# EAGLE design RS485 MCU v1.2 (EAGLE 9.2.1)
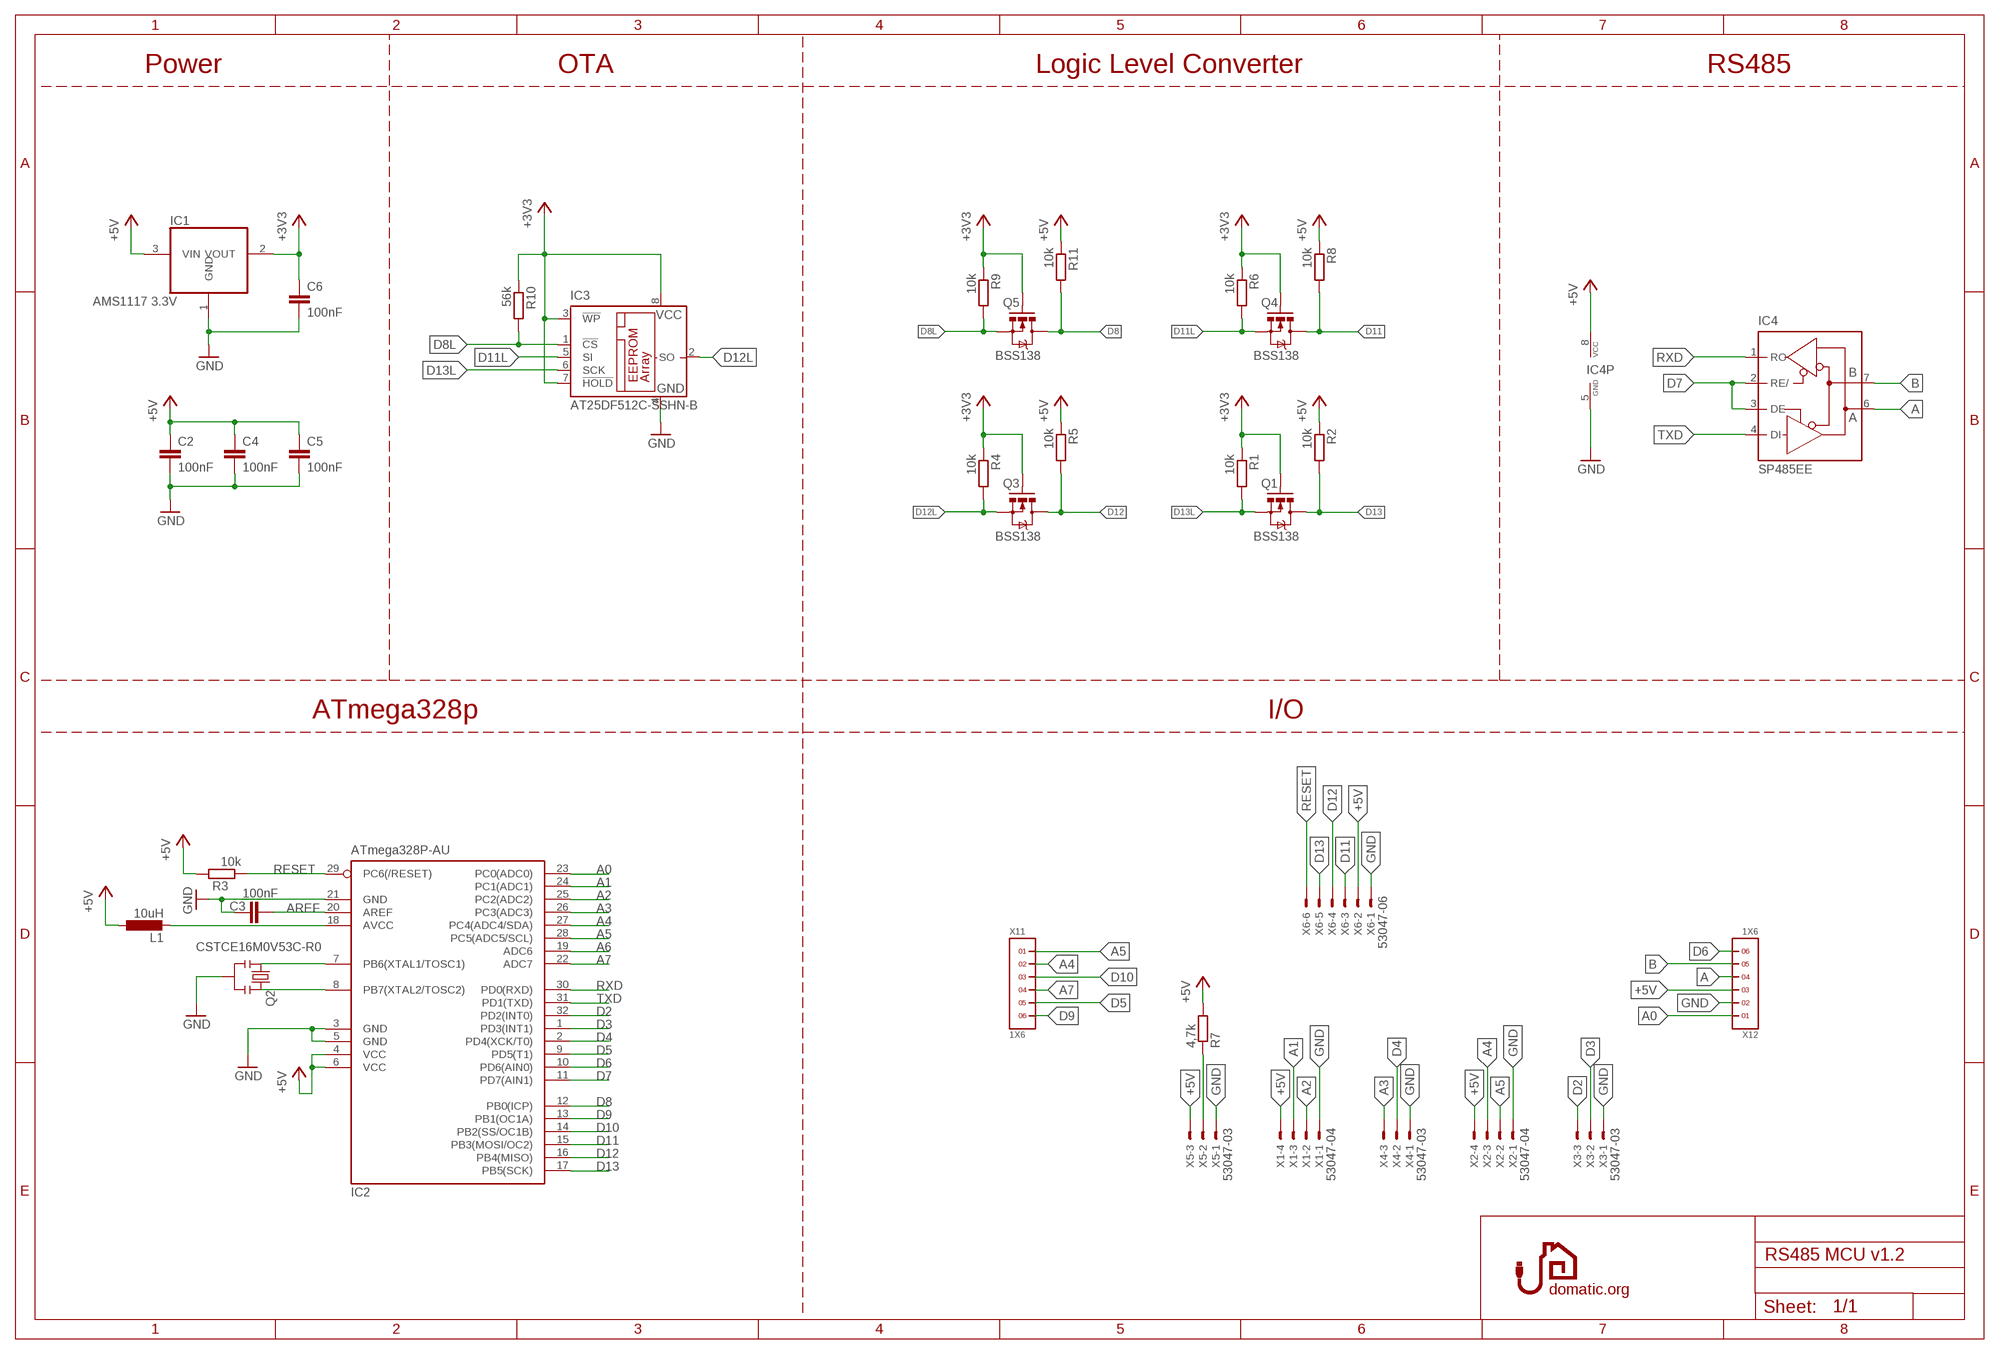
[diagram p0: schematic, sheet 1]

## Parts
C2  100nF  C-EUC0603  [C0603]
C3  100nF  C-EUC0603  [C0603]
C4  100nF  C-EUC0603  [C0603]
C5  100nF  C-EUC0603  [C0603]
C6  100nF  C-EUC0603  [C0603]
IC1  AMS1117 3.3V  REG1117  [SOT223]
IC2  ATmega328P-AU  MEGA8MEGA328P-AU-AI  [TQFP32-08]
IC3  AT25DF512C-SSHN-B  25AA080SN  [SO-08]
IC4  SP485EE  MAX481CSA  [SO08]
L1  10uH  L-EU0603  [C1608]
Q1  BSS138  MOSFET-NCHANNELSMD  [SOT23-3]
Q2  CSTCE16M0V53C-R0  RESONATOR_CSTCE_V_C  [CSTCE_V_C]
Q3  BSS138  MOSFET-NCHANNELSMD  [SOT23-3]
Q4  BSS138  MOSFET-NCHANNELSMD  [SOT23-3]
Q5  BSS138  MOSFET-NCHANNELSMD  [SOT23-3]
R1  10k  R-EU_R0603  [R0603]
R2  10k  R-EU_R0603  [R0603]
R3  10k  R-EU_R0603  [R0603]
R4  10k  R-EU_R0603  [R0603]
R5  10k  R-EU_R0603  [R0603]
R6  10k  R-EU_R0603  [R0603]
R7  4,7k  R-EU_R0603  [R0603]
R8  10k  R-EU_R0603  [R0603]
R9  10k  R-EU_R0603  [R0603]
R10  56k  R-EU_R0603  [R0603]
R11  10k  R-EU_R0603  [R0603]
X1  53047-04  [53047-04]
X2  53047-04  [53047-04]
X3  53047-03  [53047-03]
X4  53047-03  [53047-03]
X5  53047-03  [53047-03]
X6  53047-06  [53047-06]
X11  1X6  [1X6]
X12  1X6  [1X6]

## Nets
+3V3 [zasilanie]: C6.1 IC1.2(VOUT) IC3.3(!WP) IC3.7(!HOLD) IC3.8(VCC) Q1.1(G) Q3.1(G) Q4.1(G) Q5.1(G) R1.1 R4.1 R6.1 R9.1 R10.1
+5V [zasilanie]: C2.2 C4.1 C5.1 IC1.3(VIN) IC2.4(VCC) IC2.6(VCC) IC4.8(VCC) L1.1 R2.1 R3.2 R5.1 R7.2 R8.1 R11.1 X1.4 X2.4 X5.3 X6.2 X12.3
A: IC4.6(A) X12.4
A0: IC2.23(PC0(ADC0)) X12.1
A1: IC2.24(PC1(ADC1)) X1.3
A2: IC2.25(PC2(ADC2)) X1.2
A3: IC2.26(PC3(ADC3)) X4.3
A4: IC2.27(PC4(ADC4/SDA)) X2.3 X11.2
A5: IC2.28(PC5(ADC5/SCL)) X2.2 X11.1
A6: IC2.19(ADC6) R7.1 X5.2
A7: IC2.22(ADC7) X11.4
AREF: C3.2 IC2.20(AREF)
B: IC4.7(B) X12.5
D2: IC2.32(PD2(INT0)) X3.3
D3: IC2.1(PD3(INT1)) X3.2
D4: IC2.2(PD4(XCK/T0)) X4.2
D5: IC2.9(PD5(T1)) X11.5
D6: IC2.10(PD6(AIN0)) X12.6
D7: IC2.11(PD7(AIN1)) IC4.2(RE/) IC4.3(DE)
D8: IC2.12(PB0(ICP)) Q5.3(D) R11.2
D8L: IC3.1(!CS) Q5.2(S) R9.2 R10.2
D9: IC2.13(PB1(OC1A)) X11.6
D10: IC2.14(PB2(SS/OC1B)) X11.3
D11: IC2.15(PB3(MOSI/OC2)) Q4.3(D) R8.2 X6.3
D11L: IC3.5(SI) Q4.2(S) R6.2
D12: IC2.16(PB4(MISO)) Q3.3(D) R5.2 X6.4
D12L: IC3.2(SO) Q3.2(S) R4.2
D13: IC2.17(PB5(SCK)) Q1.3(D) R2.2 X6.5
D13L: IC3.6(SCK) Q1.2(S) R1.2
GND [zasilanie]: C2.1 C3.1 C4.2 C5.2 C6.2 IC1.1(GND) IC2.3(GND) IC2.5(GND) IC2.21(GND) IC3.4(GND) IC4.5(GND) Q2.GND X1.1 X2.1 X3.1 X4.1 X5.1 X6.1 X12.2
N$2: IC2.7(PB6(XTAL1/TOSC1)) Q2.X1
N$3: IC2.8(PB7(XTAL2/TOSC2)) Q2.X2
N$4 [zasilanie]: IC2.18(AVCC) L1.2
RESET: IC2.29(PC6(/RESET)) R3.1 X6.6
RXD: IC2.30(PD0(RXD)) IC4.1(RO)
TXD: IC2.31(PD1(TXD)) IC4.4(DI)

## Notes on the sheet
- Power | OTA | Logic Level Converter | RS485
- ATmega328p | I/O

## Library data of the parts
C2-C6 = resistor:C-EU: CAPACITOR, European symbol
IC1 = burr-brown:REG1117: 800mA and 1A Low Dropout (LDO) Positive Regulator 1.8V, 2.5V, 2.85V, 3.3V, 5V, and Adj; MPN: REG1117; OC_FARNELL: 1097566; OC_NEWARK: 14P6981
IC2 = atmel_2:MEGA8: MICROCONTROLLER 8 Kbytes FLASH, 1 kbytes SRAM, 512 bytes EEPROM, USART, 6-channel 10 bit ADC, 2-channel 8 bit ADC Pin compatible with Atmega48, ATMega88, ATMega168 Source: avr.lbr; MPN: ATMEGA328P-AU; SPICEPREFIX: X
IC3 = microchip:25*: Serial EEPROM 4K/ 8K , SPI bus; MF: MICROCHIP; MPN: 25AA080/SN; OC_FARNELL: 1816072; OC_NEWARK: 92C7351
IC4 = maxim:MAX481CSA: RS485 TRANSEIVER; MF: MAXIM; MPN: MAX481CSA; OC_FARNELL: unknown; OC_NEWARK: 90C3817
L1 = resistor:L-EU: INDUCTOR, European symbol
Q1 Q3-Q5 = SparkFun:MOSFET-NCHANNEL
Q2 = bt_crystal:RESONATOR: Crystal Resonator, 3-pin
R1-R11 = resistor:R-EU_: RESISTOR, European symbol
X1 X2 = con-molex:53?-04: CONNECTOR wire to board 1.25 mm (.049 inch) pitch header; MF: WALDOM/MOLEX; MPN: 53047-0410; OC_FARNELL: 9733060; OC_NEWARK: 38C9900
X3-X5 = con-molex:53?-03: CONNECTOR wire to board 1.25 mm (.049 inch) pitch header; MPN: 530470310; OC_FARNELL: 9732853; OC_NEWARK: 14R5412
X6 = con-molex:53?-06: CONNECTOR wire to board 1.25 mm (.049 inch) pitch header; MPN: 53047-0610-C; OC_FARNELL: 9733078; OC_NEWARK: 03M2965
X11 X12 = headers(2mm):1X6

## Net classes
0 default: width 0.25 mm, drill 0.5 mm, clearance 0.25 mm
1 zasilanie: width 0.3 mm, drill 0.5 mm, clearance 0.25 mm
2 230v: width 1.5 mm, drill 1 mm, clearance 2 mm

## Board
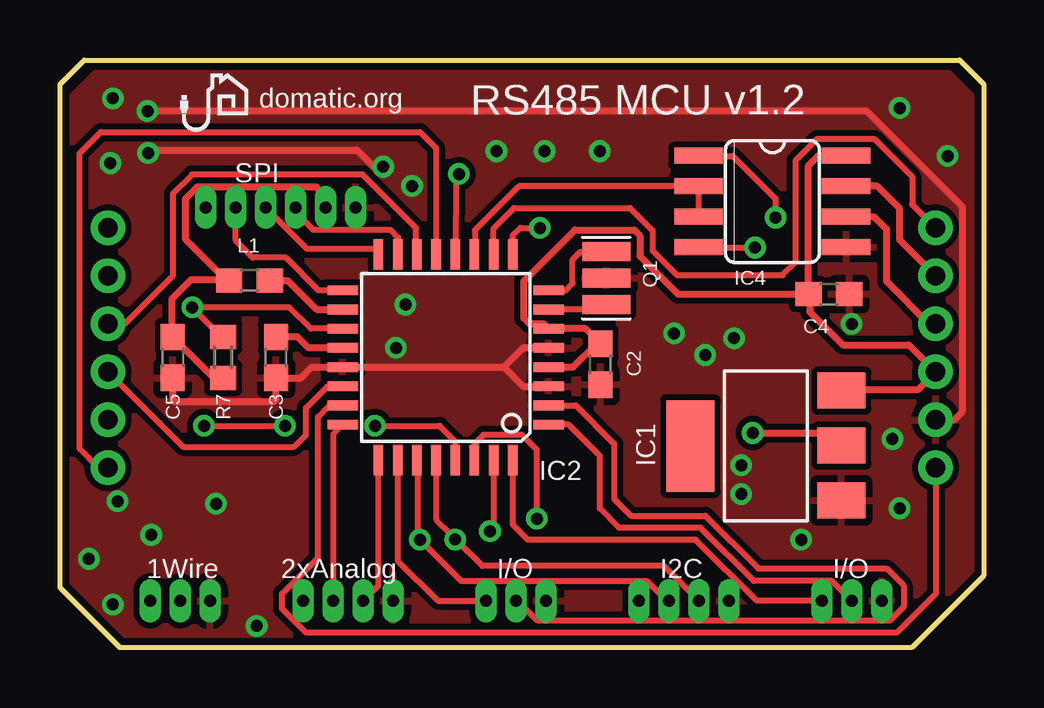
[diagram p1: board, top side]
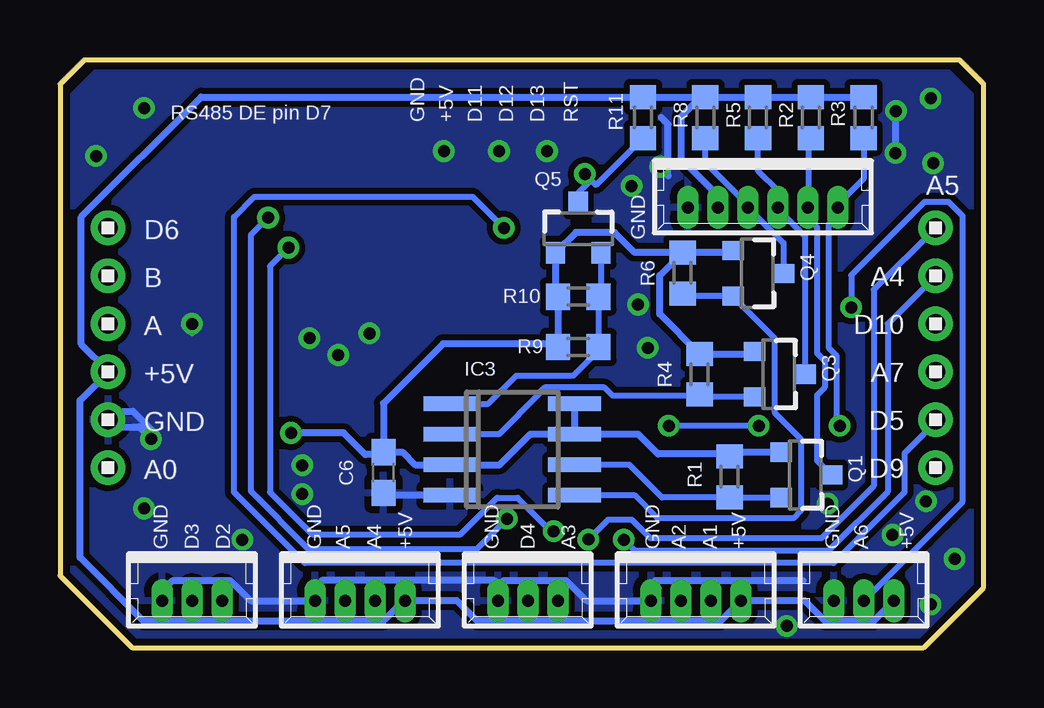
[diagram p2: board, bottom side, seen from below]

Size 38.5 x 24.5 mm. Coordinates in mm from the lower left corner, seen from the top.
Outline: 1,24.5 37.5,24.5 38.5,23.5 38.5,3 35.5,0 2.5,0 0,2.5 0,23.5 1,24.5
Copper layers (1*16): Top 0.035mm / dielectric 1.5mm / Bottom 0.035mm
Design rules "default *": minimum track width 0.15mm, minimum drill 0.5mm, track to track 0.1mm, track to pad 0.1mm, pad to pad 0.1mm, via to via 0.1mm, smd to smd 0.1mm, copper to edge 0.3mm, drill to drill 0.2mm, minimum pad ring 0.2mm, minimum via ring 0.2mm, stop-mask expansion 4mil, vias tented up to drill 0.5mm, thermal gap 0.3mm

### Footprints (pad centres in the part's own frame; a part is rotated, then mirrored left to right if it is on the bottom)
C0603 = smd 1.1 x 1: 1 -0.85,0; 2 0.85,0
SOT223 = smd 1.499 x 2.007: 1 -2.261,-3.15; 2 0.025,-3.15; 3 2.311,-3.15 | smd 3.81 x 2.007: 4 0,3.15
TQFP32-08 = smd 1.27 x 0.4: 1 -4.293,2.8; 2 -4.293,2; 3 -4.293,1.2; 4 -4.293,0.4; 5 -4.293,-0.4; 6 -4.293,-1.2; 7 -4.293,-2; 8 -4.293,-2.8; 17 4.293,-2.8; 18 4.293,-2; 19 4.293,-1.2; 20 4.293,-0.4; 21 4.293,0.4; 22 4.293,1.2; 23 4.293,2; 24 4.293,2.8 | smd 0.4 x 1.27: 9 -2.8,-4.293; 10 -2,-4.293; 11 -1.2,-4.293; 12 -0.4,-4.293; 13 0.4,-4.293; 14 1.2,-4.293; 15 2,-4.293; 16 2.8,-4.293; 25 2.8,4.293; 26 2,4.293; 27 1.2,4.293; 28 0.4,4.293; 29 -0.4,4.293; 30 -1.2,4.293; 31 -2,4.293; 32 -2.8,4.293
SO-08 = smd 0.6 x 2.2: 1 -1.905,-2.6; 2 -0.635,-2.6; 3 0.635,-2.6; 4 1.905,-2.6; 5 1.905,2.6; 6 0.635,2.6; 7 -0.635,2.6; 8 -1.905,2.6
SO08 = smd 0.66 x 2.032: 1 -1.905,-3.073; 2 -0.635,-3.073; 3 0.635,-3.073; 4 1.905,-3.073; 5 1.905,3.073; 6 0.635,3.073; 7 -0.635,3.073; 8 -1.905,3.073
C1608 = smd 1.1 x 1: 1 -0.85,0; 2 0.85,0
SOT23-3 = smd 0.8 x 0.9: 1 -0.95,-1; 2 0.95,-1; 3 0,1.1
CSTCE_V_C = smd 0.8 x 2: GND 0,0; X1 -1.1,0; X2 1.1,0
R0603 = smd 1 x 1.1: 1 -0.85,0; 2 0.85,0
53047-04 = drill 0.5 pad 0.698 long: 1 1.875,0.45; 2 0.625,0.45; 3 -0.625,0.45; 4 -1.875,0.45
53047-03 = drill 0.5 pad 0.698 long: 1 1.25,0.45; 2 0,0.45; 3 -1.25,0.45
53047-06 = drill 0.5 pad 0.698 long: 1 3.125,0.45; 2 1.875,0.45; 3 0.625,0.45; 4 -0.625,0.45; 5 -1.875,0.45; 6 -3.125,0.45
1X6 = drill 0.8 pad 1.422: 1 -5,0; 2 -3,0; 3 -1,0; 4 1,0; 5 3,0; 6 5,0

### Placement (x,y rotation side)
C2  22.53,11.81 90 top
C3  9,12.1 90 top
C4  32.05,14.73 0 top
C5  4.7,12.1 270 top
C6  25.02,7.3 270 bottom
IC1  29.43,8.4 90 top
IC2  16.08,12.1 180 top
IC3  19.65,8.26 270 bottom
IC4  29.7,18.6 270 top
L1  7.9,15.3 0 top
Q1  7.44,7.2 270 bottom
Q2  22.77,15.41 90 top
Q3  8.54,11.4 270 bottom
Q4  9.44,15.6 270 bottom
Q5  16.9,17.46 0 bottom
R1  10.59,7.12 270 bottom
R2  7.2,22.1 270 bottom
R3  5,22.1 90 bottom
R4  11.84,11.4 270 bottom
R5  9.4,22.1 270 bottom
R6  12.55,15.62 270 bottom
R7  6.8,12.1 270 top
R8  11.6,22.1 270 bottom
R9  16.9,12.53 0 bottom
R10  16.9,14.63 0 bottom
R11  14.2,22.1 270 bottom
U$3  [LOGO2.5MMNAP0,8]  5,21.5 0 top
X1  12,2.4 180 bottom
X2  26,2.4 180 bottom
X3  33,2.4 180 bottom
X4  19,2.4 180 bottom
X5  5,2.4 180 bottom
X6  9.2,18.8 180 bottom
X11  2,12.5 270 bottom
X12  36.5,12.5 90 bottom

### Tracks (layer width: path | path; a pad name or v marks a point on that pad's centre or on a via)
+3V3  (via drill 0.5)
  Top 0.3: v28.88,8.95 31.57,8.95 32.02,8.5 32.5,8.5 IC1.2 32.62,8.38 IC1.2
  Bottom 0.3: Q4.1 10.52,16.47 R6.1 | IC3.7 14.39,8.89 13.57,8.07 10.69,8.07 R1.1 10.41,8.15 Q1.1 | Q3.1 9.64,12.25 R4.1 13.5,13.9 13.5,15.52 R6.1 | R6.1 14.54,16.47 15.38,17.31 17,17.31 Q5.1 17.85,14.73 R10.1 R9.1 17.89,12.66 22.54,12.66 25.02,10.18 C6.1 | IC3.8 IC3.7 | IC3.7 18.91,8.89 20.18,7.62 IC3.3 | 22.23,7.6 IC3.3 | C6.1 24.22,8.15 23.7,7.62 IC3.3 | C6.1 25.02,8.05 25.77,8.05 26.68,8.95 v28.88,8.95
+5V
  Top 0.3: IC2.4 21.4,11.7 22.36,12.66 C2.2 | C2.2 21.9,13.3 20.5,13.3 | 20.5,13.3 IC2.6 | IC2.6 20.17,13.5 19.57,13.5 19.34,13.73 19.34,15.28 21.46,17.41 23.94,17.41 24.17,17.17 24.17,16.33 25.77,14.73 C4.1 | C4.1 31.2,20.1 31.61,20.5 IC4.8 | X6.2 11.03,18.85 10.68,19.2 5.72,19.2 5.22,18.7 5.22,17.03 6.96,15.3 L1.1 7.02,15.33 5.46,15.33 4.67,14.54 4.67,12.98 C5.1 6.4,11.25 R7.2 | 32.62,10.75 35.75,10.75 X12.3 35.38,12.62 32.62,12.62 31.25,14 31.26,14.62 | 32.62,10.75 IC1.3 | 31.26,14.62 31.26,14.64 31.19,14.72 | C2.2 | 22.62,12.75 C2.2 | 20.5,13.3 20.5,13.38 IC2.6 | 32.62,10.75 IC1.3 | 31.26,14.62 31.12,14.62 C4.1 | IC2.6
  Bottom 0.3: X5.3 4.6,1.1 6.6,1.1 7.45,1.95 X1.4 10.97,1.1 21.1,1.1 21.95,1.95 X2.4 24.17,1.95 25.02,1.1 35,1.1 37.66,3.76 37.66,10.31 36.5,11.47 X12.3 36.5,11.53 37.61,12.64 37.61,17.96 32.62,22.95 R11.1 11.8,22.95 | 11.8,22.95 R8.1 R5.1 R2.1 R3.2 | 11.8,22.95 12.6,22.15 12.6,20.38 11.07,18.85 X6.2
A
  Top 0.3: IC4.6 33.94,17.96 34.45,17.45 34.45,15.28 36.23,13.5 X12.4
A0
  Top 0.25: IC2.23 11.22,10.1 10.75,9.62 10.75,3.75 9.25,2.25 9.25,1.62 10.25,0.62 34.88,0.62 36.5,2.25 X12.1 | IC2.23 | IC2.23 | IC2.23 11.88,10.12 IC2.23
A1
  Top 0.25: X1.3 11.39,1.96 11.39,8.9 IC2.24
A2
  Top 0.25: X1.2 13.28,2.6 IC2.25
A3
  Top 0.25: IC2.26 14.08,3.62 15.75,1.95 X4.3
A4  (via drill 0.5)
  Top 0.25: 25.29,1.95 X2.3 | X2.3 | 25.29,1.95 24.47,2.77 16.73,2.77 v15,4.5 14.9,4.6 14.9,7.68 14.88,7.7 IC2.27 | X2.3 25.38,2 25.29,1.95
  Bottom 0.25: X11.2 4,13.5 4,6.5 6.47,4.03 14.53,4.03 v15,4.5
A5  (via drill 0.5)
  Top 0.25: X2.2 25.18,3.4 17.61,3.4 16.48,4.53 | IC2.28 15.7,7.78 15.7,5.3 16.25,4.75 | 16.25,4.75 16.34,4.67 16.48,4.53 | 16.48,4.53 v16.48,4.5 16.25,4.75
  Bottom 0.25: X11.1 4.58,14.93 4.58,6.73 6.75,4.55 13.89,4.55 14.66,5.33 15.65,5.33 v16.48,4.5 | v16.48,4.5 | 16.5,4.5 v16.48,4.5
A6  (via drill 0.5)
  Top 0.25: IC2.19 10.46,13.3 9.57,14.18 v5.51,14.18 6.75,12.95 R7.1
  Bottom 0.25: v5.51,14.18 5.51,15.52 2.45,18.59 1.46,18.59 0.88,18 0.88,6.08 X5.2
A7
  Top 0.25: 11.75,10.87 11.12,10.88 10.25,10 10.25,8.88 9.75,8.38 5.12,8.38 X11.4 | 11.75,10.87 IC2.22 | IC2.22 11.88,10.88 11.75,10.87
AREF
  Top 0.3: IC2.20 10.35,12.5 9.9,12.95 C3.2
B
  Top 0.3: X12.5 35,17 35,18.3 34.06,19.23 IC4.7
D2
  Top 0.25: X3.3 29.04,1.95 26.49,4.5 19.5,4.5 18.88,5.12 IC2.32 | X3.3 | 31.75,2 X3.3
D3
  Top 0.25: X3.2 32.17,2.77 28.92,2.77 26.7,5 23.3,5 22.5,5.8 22.5,8 21.2,9.3 IC2.1
D4
  Top 0.25: 19.08,1.95 X4.2 | X4.2 | 19.08,1.95 19.91,1.12 34.59,1.12 35.17,1.71 35.17,2.59 34.47,3.3 29.11,3.3 26.91,5.5 23.8,5.5 23.1,6.2 23.1,8.5 21.5,10.1 IC2.2 | X4.2 19,2 19.08,1.95
D5  (via drill 0.5)
  Top 0.25: v20,17.5 19.19,17.5 18.88,17.19 IC2.9
  Bottom 0.25: X11.5 2,9.4 3.3,8.1 3.3,6.47 6.25,3.53 28.3,3.53 31.25,6.47 31.25,17.95 30.4,18.8 21.3,18.8 v20,17.5
D6
  Top 0.25: IC2.10 18.08,17.48 18.93,18.32 23.76,18.32 24.7,17.39 24.7,16.54 25.72,15.52 30.12,15.52 30.68,16.07 30.68,20.32 31.57,21.21 33.95,21.21 35.52,19.63 35.52,18.48 X12.6
D7
  Top 0.25: IC4.3 IC4.2 19.13,19.23 17.58,17.69 17.58,17.68 17.3,17.4 17.3,16.41 IC2.11
D8  (via drill 0.5)
  Top 0.25: v16.62,19.75 16.5,19.62 16.49,16.5 IC2.12 16.5,16.38 IC2.12
  Bottom 0.25: R11.2 16.16,19.29 16.36,19.49 | 16.36,19.49 16.9,18.95 Q5.3 | 16.36,19.49 v16.62,19.75
D8L
  Bottom 0.25: Q5.2 15.95,14.73 R10.2 R9.2 16.05,12.39 17.1,11.34 19.48,11.34 20.65,10.16 IC3.1
D9
  Top 0.25: X11.6 1.6,7.5 0.82,8.28 0.82,20.62 1.7,21.5 15,21.5 15.68,20.82 IC2.13
D10
  Top 0.25: IC2.14 14.85,16.41 14.85,17.49 12.62,19.73 5.5,19.73 4.7,18.92 4.7,15.5 2.7,13.5 X11.3
D11
  Top 0.25: X6.3 9.82,18.15 10.55,17.43 13.78,17.43 14.1,17.1 14.08,17.08 IC2.15
  Bottom 0.25: Q4.3 8.34,16.86 X6.3 9.82,18.45 11.6,20.23 R8.2
D11L
  Bottom 0.25: R6.2 12.43,14.65 Q4.2 10.44,14.63 8.71,12.9 8.71,9.8 7.62,8.71 7.62,5.7 7.92,5.39 13.6,5.39 14.55,6.36 IC3.5 | IC3.5 | 17.12,6.38 IC3.5
D12
  Top 0.25: X6.4 | X6.4 8.57,18.25 | X6.4 10.3,16.62 13.28,16.62 IC2.16
  Bottom 0.25: Q3.3 7.44,17.15 8.57,18.29 X6.4 8.57,19.05 9.4,19.88 R5.2
D12L
  Bottom 0.25: Q3.2 11.74,10.45 R4.2 11.89,10.5 15.46,10.5 15.79,10.84 18.3,10.84 18.52,10.62 18.52,10.57 20.2,8.89 IC3.2
D13
  Top 0.25: IC2.17 10.78,14.9 9.42,16.26 8.04,16.26 7.33,16.98 X6.5
  Bottom 0.25: R2.2 7.3,21.15 7.3,18.48 X6.5 7.33,17.91 6.94,17.52 6.94,12.28 6.62,11.96 6.62,10.85 6.94,10.52 6.94,7.8 Q1.3
D13L
  Bottom 0.25: Q1.2 8.46,6.27 R1.2 10.61,6.25 13.4,6.25 14.77,7.62 IC3.6
GND  (via drill 0.5)
  Top 0.3: C5.2 4.7,10.35 4.8,10.25 8.9,10.25 9,10.35 C3.1 10.05,11.25 10.5,11.7 IC2.21 18.5,11.7 | IC2.3 19.3,10.9 18.5,11.7 | IC2.5 19.3,12.5 18.5,11.7 | 33,14.63 C4.2 32.88,14.75 C4.2 | v13.47,20.05 13.07,20.05 12.38,20.75 3.8,20.75 v3.67,20.62 | v3.65,22.38 33.62,22.38 37.62,18.38 37.62,9.85 37.27,9.5 X12.2
  Bottom 0.3: 7.52,2.8 13.68,2.8 13.88,2.6 X1.1 16.55,1.95 17.4,2.8 20,2.8 20.25,2.55 X4.1 20.25,2.65 20.4,2.8 27.58,2.8 27.88,2.5 X2.1 30.55,1.95 31.4,2.8 33.8,2.8 34.25,2.35 X3.1 | 13.15,19.68 13.15,20.05 | 13.15,20.05 13.15,21.82 13.43,22.1 | C6.2 24.93,6.36 IC3.4 | 33,13.12 v33,13.5 | v13.47,20.05 13.15,20.05 | v3.65,22.38 3.67,22.35 v3.67,20.62 | 35.45,9.85 34.7,9.1 v34.7,8.7 35.2,9.2 36.2,9.2 X12.2 36.15,9.85 35.45,9.85
  other vias: 35,22.5 37,20.5 20.2,20.7 14,12.5 14.4,14.3 6.5,6 26.9,12.2 2.4,6.1 30.9,4.5 35,5.8 18.2,20.7 22.5,20.7 2.1,20.2 2.2,22.9 8.2,0.9 3.8,4.7 25.6,13.1 28.1,12.9 28.4,7.6 28.4,6.4 14.68,19.25 2.2,1.8 1.2,3.7
  pour Top (isolate 0.25): 36.5,24.5 2,24.5 0,22.5 0,3 2.5,0.5 36,0.5 38.5,3 38.5,22.5
  pour Bottom (isolate 0.25): 36.5,24.5 2,24.5 0,22.5 0,3 2.5,0.5 36,0.5 38.5,3 38.5,22.5
N$2
  Top 0.25: IC2.7 22.06,14.1 22.27,14.31 Q2.X1
N$3
  Top 0.25: Q2.X2 21.71,16.51 21.37,16.17 21.37,15.2 21.07,14.9 IC2.8
N$4
  Top 0.3: IC2.18 10.7,14.1 9.5,15.3 L1.2 | IC2.18
RESET  (via drill 0.5)
  Top 0.25: 16.48,7.87 16.48,8.6 15.82,9.25 v13.12,9.25 | 16.48,7.87 IC2.29 16.5,7.88 16.48,7.87 | v6,9.25 v9.38,9.25
  Bottom 0.25: v9.38,9.25 v13.12,9.25 | R3.1 5,19.55 6.08,18.48 X6.6 6.08,18 6.44,17.64 6.44,12.49 6.12,12.16 6.12,9.37 v6,9.25
RXD  (via drill 0.5)
  Top 0.25: v19.88,5.38 19.88,8.25 19.25,8.88 17.65,8.88 17.27,8.5 IC2.30 | v29.82,17.93 29.82,18.73 28.05,20.5 26.75,20.5 IC4.1
  Bottom 0.25: v19.88,5.38 21.12,4.12 28.15,4.12 30.55,6.53 30.55,17.2 v29.82,17.93
TXD  (via drill 0.5)
  Top 0.25: v17.93,4.85 18.07,5 IC2.31 18.13,7.75 18.12,7.88 IC2.31 | 26.75,16.68 26.66,16.68 IC4.4 | 26.75,16.68 v28.98,16.68 | 26.75,16.68 26.75,16.62 IC4.4
  Bottom 0.25: v17.93,4.85 18.02,4.85 19.43,6.25 20.27,6.25 21.8,4.72 28,4.72 29.75,6.47 29.75,15.9 v28.98,16.68

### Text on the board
tNames: RS485 MCU v1.2 | SPI | Q1 | 1Wire | 2xAnalog | I/O | I2C | I/O
bNames: RS485 DE pin D7 | RST | D13 | D12 | D11 | +5V | GND | A5 | GND | D6 | A4 | B | D10 | A | A7 | +5V | D5 | GND | D9 | A0 | +5V | A6 | GND | +5V | A1 | A2 | GND | A3 | D4 | GND | +5V | A4 | A5 | GND | D2 | D3 | GND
